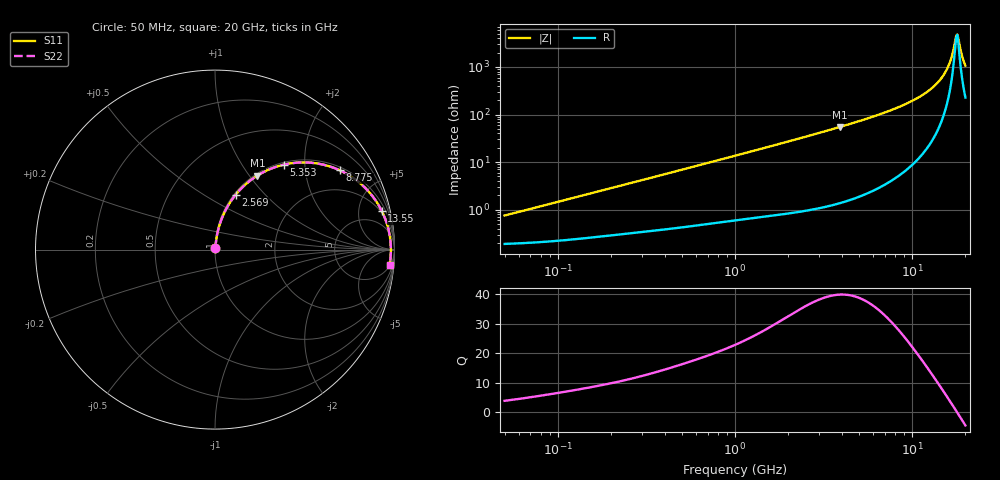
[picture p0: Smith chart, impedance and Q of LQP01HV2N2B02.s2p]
!Murata Part Number: LQP01HV2N2B02
!These Parameters are Measured in Series Mode Connection
!  o--[Z]--o
!Port1  Port2
!  o-------o
!Freq. Start=50[MHz] Stop=20[GHz], 401[Steps]
# Hz S RI R 50
!Freq.(Hz) S11(Real) S11(Imag) S21(Real) S21(Imag) S12(Real) S12(Imag) S22(Real) S22(Imag)
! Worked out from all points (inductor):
!   401 points, 50 MHz to 20 GHz, reference 50 ohm
!   read as one part in series: L = 2.32 nH near 51.52 MHz
!   highest Q = 40 at 3.908 GHz (marker M1), where L = 2.23 nH
!   self-resonance near 17.74 GHz
!   S11 on the Smith chart (normalised r, x): 50 MHz: 1.00, +0.01; 2.569 GHz: 1.02, +0.70; 5.353 GHz: 1.04, +1.57; 8.775 GHz: 1.12, +3.07; 13.55 GHz: 1.75, +8.35; 20 GHz: 6, -21
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5e7  0.00195 0.00727  0.998 -0.00727  0.998 -0.00727  0.00195 0.00727
1.364002e8  0.00285 0.0194  0.9972 -0.0194  0.9972 -0.0194  0.00285 0.0194
3.721004e8  0.00633 0.0511  0.9937 -0.0511  0.9937 -0.0511  0.00633 0.0511
1e9  0.0237 0.1318  0.9763 -0.1318  0.9763 -0.1318  0.0237 0.1318
1.714689e9  0.0576 0.2171  0.9424 -0.2171  0.9424 -0.2171  0.0576 0.2171
2.569357e9  0.1161 0.3069  0.8839 -0.3069  0.8839 -0.3069  0.1161 0.3069
2.728004e9  0.1287 0.3217  0.8713 -0.3217  0.8713 -0.3217  0.1287 0.3217
3.908127e9  0.236 0.4123  0.764 -0.4123  0.764 -0.4123  0.236 0.4123
5.352748e9  0.383 0.4732  0.617 -0.4732  0.617 -0.4732  0.383 0.4732
7.442007e9  0.5863 0.4768  0.4137 -0.4768  0.4137 -0.4768  0.5863 0.4768
8.774992e9  0.6955 0.4417  0.3045 -0.4417  0.3045 -0.4417  0.6955 0.4417
1.131968e10  0.8489 0.3312  0.1511 -0.3312  0.1511 -0.3312  0.8489 0.3312
1.354865e10  0.9287 0.2162  0.0713 -0.2162  0.0713 -0.2162  0.9287 0.2162
1.482269e10  0.9558 0.1501  0.0442 -0.1501  0.0442 -0.1501  0.9558 0.1501
1.573793e10  0.9685 0.1038  0.0315 -0.1038  0.0315 -0.1038  0.9685 0.1038
1.646126e10  0.975 0.0684  0.025 -0.0684  0.025 -0.0684  0.975 0.0684
1.747767e10  0.9795 0.0204  0.0205 -0.0204  0.0205 -0.0204  0.9795 0.0204
1.774144e10  0.9799 0.00839  0.0201 -0.00839  0.0201 -0.00839  0.9799 0.00839
1.800918e10  0.98 -0.00366  0.02 0.00366  0.02 0.00366  0.98 -0.00366
1.828096e10  0.9798 -0.0157  0.0202 0.0157  0.0202 0.0157  0.9798 -0.0157
1.940974e10  0.976 -0.0638  0.024 0.0638  0.024 0.0638  0.976 -0.0638
2e10  0.9723 -0.0876  0.0277 0.0876  0.0277 0.0876  0.9723 -0.0876
